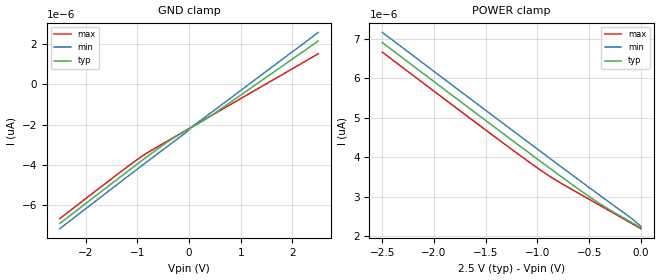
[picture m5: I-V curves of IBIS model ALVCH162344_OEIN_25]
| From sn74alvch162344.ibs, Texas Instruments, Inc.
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[Model]   ALVCH162344_OEIN_25
Model_type  Input
Vinl = 0.7
Vinh = 1.7
| variable   typ   min   max
C_comp   1.28pF   1.14pF   1.41pF
[Temperature Range]   40   100   -40
| Ambient temperature   25   85   -40
[Voltage range]   2.5   2.3   2.7
[GND Clamp]
| ALVCH162344_OEIN_25
|   Voltage   I(typ)   I(min)   I(max)
-2.5V     -6.898pA   -7.156pA   -6.656pA
-1.29V    -4.513pA   -4.769pA   -4.274pA
-850mV    -3.658pA   -3.907pA   -3.461pA
-365mV    -2.767pA   -2.969pA   -2.73pA
440mV     -1.528pA   -1.373pA   -1.532pA
2.5V      2.157pA    2.582pA    1.524pA
[POWER Clamp]
| ALVCH162344_OEIN_25
|   Voltage   I(typ)   I(min)   I(max)
-2.5V     6.898pA    7.156pA    6.656pA
-1.425V   4.777pA    5.034pA    4.537pA
-950mV    3.851pA    4.102pA    3.632pA
-785mV    3.533pA    3.78pA     3.358pA
-415mV    2.851pA    3.065pA    2.804pA
-105mV    2.367pA    2.474pA    2.342pA
0V        2.211pA    2.242pA    2.186pA
